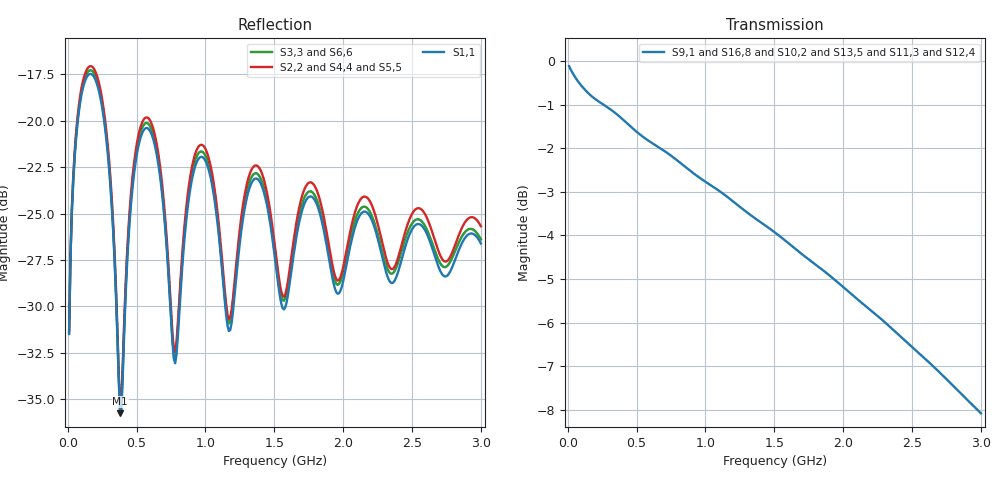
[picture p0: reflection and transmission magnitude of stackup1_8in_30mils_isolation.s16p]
! Touchstone file from project
# GHZ S RI R 50.000000
! Modal data exported
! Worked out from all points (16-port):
!   300 points, 10 MHz to 3 GHz, reference 50 ohm
!   strongest paths, dB at 10 MHz, 760 MHz, 1.51 GHz, 2.26 GHz, 3 GHz:
!     S9,1: -0.1, -2.2, -3.9, -5.9, -8.1
!     S16,8: -0.1, -2.2, -3.9, -5.9, -8.1
!     S10,2: -0.1, -2.2, -4.0, -5.9, -8.2
!     S13,5: -0.1, -2.2, -4.0, -5.9, -8.2
!     S11,3: -0.1, -2.2, -4.0, -5.9, -8.2
!     S12,4: -0.1, -2.2, -4.0, -5.9, -8.2
!   lowest |S11| = -35.8 dB at 380 MHz (marker M1), VSWR 1.03, Z = 51.5 - j0.74 ohm
!   |S11| at or under -10 dB: start of sweep to end of sweep
